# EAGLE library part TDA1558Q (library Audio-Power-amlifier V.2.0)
The TDA1558Q is a monolithic integrated class-B output amplifier in a 17-lead single-in-line (SIL) plastic power package. The device contains 4 x 11 W single-ended or 2 x 22 W BTL amplifiers and has been primarily developed for car radio applications.
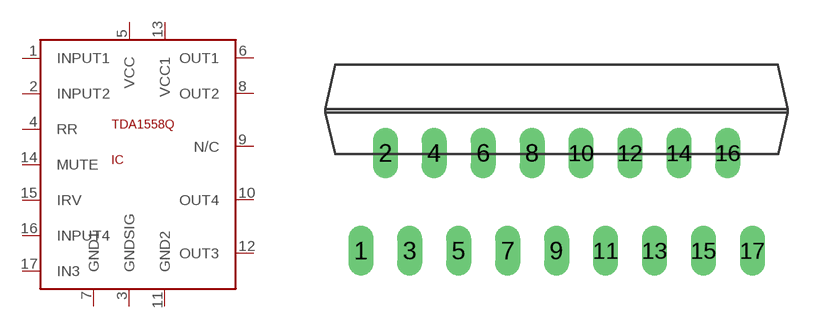
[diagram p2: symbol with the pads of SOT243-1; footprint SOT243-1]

Designator prefix IC

## TDA1558Q  [SOT243-1]
1  INPUT1  in
2  INPUT2  in
3  GNDSIG  pwr
4  RR  pas
5  VCC  pwr
6  OUT1  out
7  GND1  pwr
8  OUT2  out
9  N/C  nc
10  OUT4  out
11  GND2  pwr
12  OUT3  out
13  VCC1  pwr
14  MUTE  in
15  IRV
16  INPUT4  in
17  IN3  in

## Footprint SOT243-1 (pad centres in mm)
DBS17P: plastic DIL-bent-SIL power package; 17 leads (lead length 7.7 mm)
drill 0.8 long: 1 -10.16,-5.08; 2 -8.89,0; 3 -7.62,-5.08; 4 -6.35,0; 5 -5.08,-5.08; 6 -3.81,0; 7 -2.54,-5.08; 8 -1.27,0; 9 0,-5.08; 10 1.27,0; 11 2.54,-5.08; 12 3.81,0; 13 5.08,-5.08; 14 6.35,0; 15 7.62,-5.08; 16 8.89,0; 17 10.17,-5.08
